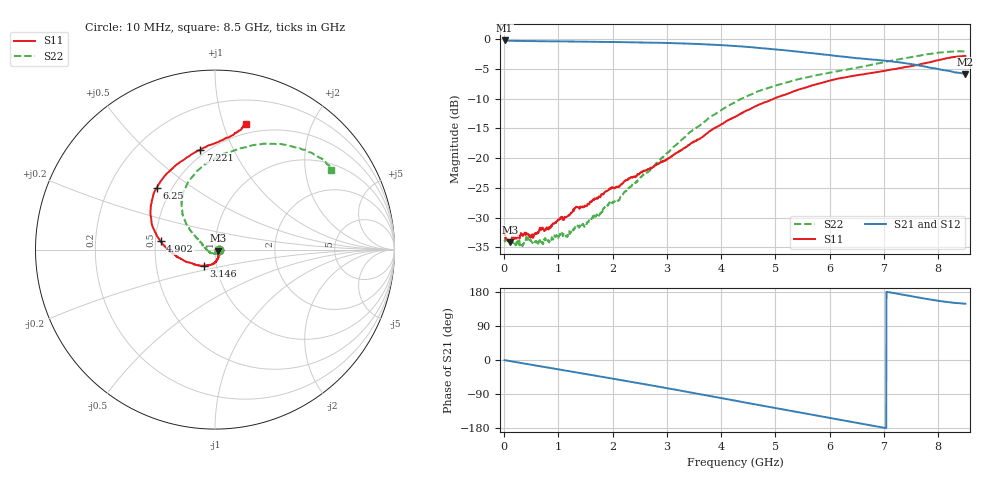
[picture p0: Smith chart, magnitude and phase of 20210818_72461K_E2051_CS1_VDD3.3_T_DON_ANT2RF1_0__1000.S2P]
!Agilent Technologies,E5071C,MY46417908,A.11.23
!Date: Wed Aug 18 14:22:55 2021
!Data & Calibration Information:
!Freq	S11:SOLT2(ON)	S21:SOLT2(ON)	S12:SOLT2(ON)	S22:SOLT2(ON)
!PortZ  Port1:50+j0  Port2:50+j0
!Above PortZ is port z conversion or system Z0 setting when saving the data.
!When reading, reference impedance value at option line is always used.
# Hz S dB R 50
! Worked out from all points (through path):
!   1601 points, 10 MHz to 8.5 GHz, reference 50 ohm
!   highest |S21| = -0.23 dB at 10 MHz (marker M1); lowest = -5.9 dB at 8.5 GHz (marker M2)
!   group delay of S21, straight-line fit = 71.1 ps
!   lowest |S11| = -34.1 dB at 110.8 MHz (marker M3), VSWR 1.04, Z = 51.9 - j0.585 ohm
!   |S11| at or under -10 dB: start of sweep to 4.976 GHz
!   |S22| runs from -34.8 to -2.0 dB; largest |S21 - S12| = 0.0042
!   S11 on the Smith chart (normalised r, x): 10 MHz: 1.05, +0.00; 3.146 GHz: 0.87, -0.16; 4.902 GHz: 0.53, +0.05; 6.25 GHz: 0.41, +0.37; 7.221 GHz: 0.46, +0.75; 8.5 GHz: 0.41, +1.19
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1e7  -32.14 0.2  -0.23 -0.4  -0.23 -0.4  -33.74 -9.7
1.108188e8  -34.13 -16.7  -0.28 -2.9  -0.27 -2.9  -34.11 -20.8
3.28375e8  -32.81 -26.3  -0.31 -8.3  -0.31 -8.3  -34.57 -47.0
4.451125e8  -32.76 -35.2  -0.32 -11.2  -0.32 -11.2  -33.42 -49.6
5.459312e8  -33.16 -39.3  -0.34 -13.6  -0.34 -13.6  -34.02 -57.8
8.271625e8  -31.86 -48.7  -0.36 -20.4  -0.36 -20.4  -34.13 -76.6
1.055331e9  -30.06 -56.6  -0.38 -26.0  -0.38 -26.0  -32.64 -94.4
1.177375e9  -29.71 -54.9  -0.40 -29.0  -0.40 -29.0  -32.91 -105.2
1.320644e9  -28.28 -60.8  -0.42 -32.5  -0.42 -32.5  -31.62 -121.6
1.426769e9  -28.29 -61.9  -0.42 -35.1  -0.43 -35.1  -31.20 -132.7
2.111275e9  -24.76 -78.8  -0.50 -51.9  -0.50 -51.9  -27.11 179.6
2.843538e9  -20.90 -108.0  -0.62 -70.4  -0.62 -70.4  -20.51 152.3
3.145994e9  -19.27 -124.0  -0.69 -78.1  -0.69 -78.1  -17.94 146.9
3.6607e9  -16.45 -150.0  -0.85 -91.6  -0.85 -91.6  -14.12 139.6
4.255e9  -13.09 -171.4  -1.16 -107.2  -1.15 -107.2  -10.62 128.5
4.902362e9  -10.28 171.3  -1.65 -124.2  -1.65 -124.2  -8.11 113.6
5.671769e9  -7.80 151.6  -2.36 -144.2  -2.38 -144.4  -6.23 94.5
6.25015e9  -6.49 133.1  -2.96 -159.1  -2.95 -159.3  -5.25 82.0
7.088538e9  -5.19 102.7  -3.69 178.9  -3.69 178.9  -3.72 64.8
7.221194e9  -5.00 98.3  -3.84 175.6  -3.84 175.5  -3.50 61.8
7.911006e9  -3.71 80.6  -4.88 158.3  -4.86 158.2  -2.38 45.3
8.5e9  -2.83 76.1  -5.90 148.5  -5.84 148.5  -2.12 34.5
